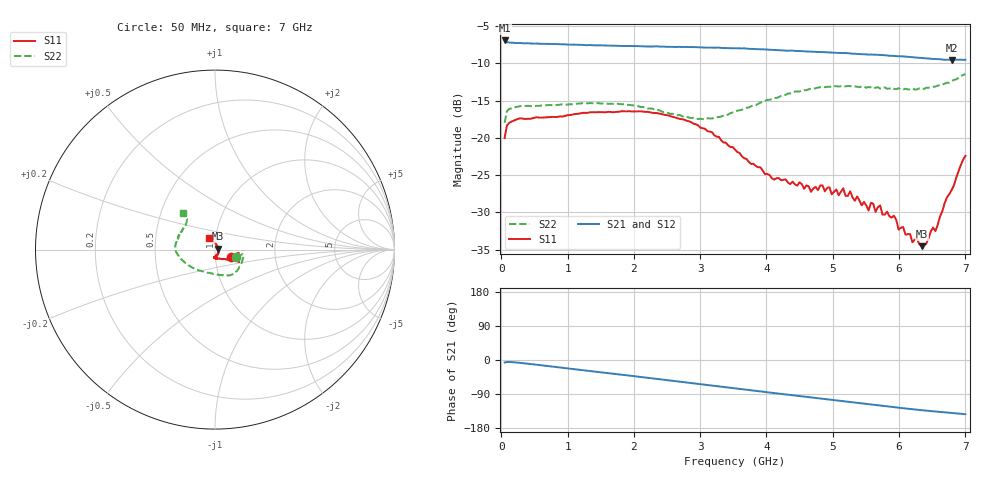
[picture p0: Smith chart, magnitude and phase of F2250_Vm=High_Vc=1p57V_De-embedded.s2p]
! Integrated Device Technology
! Corporate Headquarters
! 6024 Silver Creek Valley Road
! San Jose, CA 95138  USA
! Phone:  1-408-284-8200
! Toll Free:  1-800-223-1366
! Webpage:  http://www.idt.com/
! Timing and RF Division
! 515 Groton Road, Suite 102
! Westford, MA 01886-6024
! Device:  F2250
! Description: Voltage Variable RF Attenuator
! Frequency:  50.0 -  6000.00 MHz
! Package:  3x3 mm Thin QFN Plastic Package: 16 pin
! Ports:  2 RF, 3 DC
!  Pin  1  = GND
!  Pin  2  = NC
!  Pin  3  = RF1  = Port 1
!  Pin  4  = NC
!  Pin  5  = GND
!  Pin  6  = GND
!  Pin  7  = GND
!  Pin  8  = GND
!  Pin  9  = NC
!  Pin 10  = RF2  = Port 2
!  Pin 11  = NC
!  Pin 12  = GND
!  Pin 13  = GND
!  Pin 14  = VCNTRL
!  Pin 15  = VDD
!  Pin 16  = VMODE
! Vcntrl:  1.570 Volts
! Vmode:  +3.300 Volts
! Vdd:  +3.30  Volts
! Current:  1.330 mA
! Data:  The device was measured on a the F2250 evaluation board which has
!  individual transmission lines to the RF pins.  Data was collected
!  using a calibrated network analyzer.  The evaluation board was
!  de-embedded using a TRL calibration technique.
!  The reference plane is the edge of the package pin.
! Misc:  SN 10
!  Action Tracker AT0258
! Date Measured:  2014-11-26
! Date:  2015-10-15  MJV
! Note:
!  Integrated Device Technology supplies this data as a sample of measured
!  data at the package pin for this product.  Your particular data for this
!  product may vary.
!  Data was taken at 25 degrees C.
!  Integrated Device Technology reserves the right to change this data at anytime.
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# GHz S dB R 50
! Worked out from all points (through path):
!   201 points, 50 MHz to 7 GHz, reference 50 ohm
!   highest |S21| = -6.94 dB at 50 MHz (marker M1); lowest = -9.6 dB at 6.792 GHz (marker M2)
!   group delay of S21, straight-line fit = 57.3 ps
!   lowest |S11| = -34.5 dB at 6.34 GHz (marker M3), VSWR 1.04, Z = 51.8 + j0.574 ohm
!   |S11| at or under -10 dB: start of sweep to end of sweep
!   |S22| runs from -18.0 to -11.4 dB; largest |S21 - S12| = 0.0023
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0.05  -20.04 -25.9  -6.94 -6.6  -6.94 -6.6  -17.98 -18.7
0.08475  -18.35 -12.9  -7.16 -5.3  -7.15 -5.3  -16.41 -10.6
0.2585  -17.44 -8.9  -7.29 -7.1  -7.28 -7.1  -15.81 -12.3
1.2315  -16.65 -23.8  -7.54 -27.0  -7.56 -27.0  -15.35 -42.6
2.37825  -16.74 -27.1  -7.75 -50.4  -7.77 -50.4  -16.28 -70.9
2.969  -18.33 -28.7  -7.86 -62.8  -7.86 -62.8  -17.49 -97.7
3.525  -21.58 -40.5  -7.99 -74.7  -8.00 -74.8  -16.53 -130.8
4.11575  -25.60 -70.2  -8.21 -87.3  -8.18 -87.4  -14.66 -157.5
4.7065  -26.79 -95.5  -8.46 -99.7  -8.47 -99.7  -13.43 -174.7
5.08875  -27.71 -93.5  -8.62 -107.6  -8.61 -107.7  -13.12 176.1
5.15825  -26.78 -92.4  -8.64 -109.0  -8.63 -109.1  -13.04 174.6
5.5405  -29.75 -82.2  -8.84 -116.8  -8.83 -116.9  -13.19 164.6
5.57525  -28.72 -80.6  -8.83 -117.4  -8.82 -117.5  -13.24 164.8
5.64475  -29.94 -74.6  -8.86 -118.9  -8.84 -119.1  -13.28 161.4
5.71425  -29.07 -68.7  -8.90 -120.3  -8.88 -120.4  -13.39 160.6
5.749  -30.29 -65.8  -8.91 -121.0  -8.90 -121.2  -13.31 158.6
5.85325  -30.52 -58.9  -9.00 -123.0  -8.97 -123.2  -13.40 156.1
6.33975  -34.54 17.2  -9.28 -132.4  -9.30 -132.5  -13.45 141.5
6.5135  -32.04 62.0  -9.43 -135.4  -9.41 -135.6  -13.16 136.3
6.54825  -32.51 68.2  -9.43 -136.1  -9.43 -136.2  -13.13 135.6
6.7915  -27.02 98.8  -9.55 -139.6  -9.54 -139.8  -12.40 131.7
7  -22.43 118.4  -9.53 -143.0  -9.54 -143.2  -11.41 131.3
